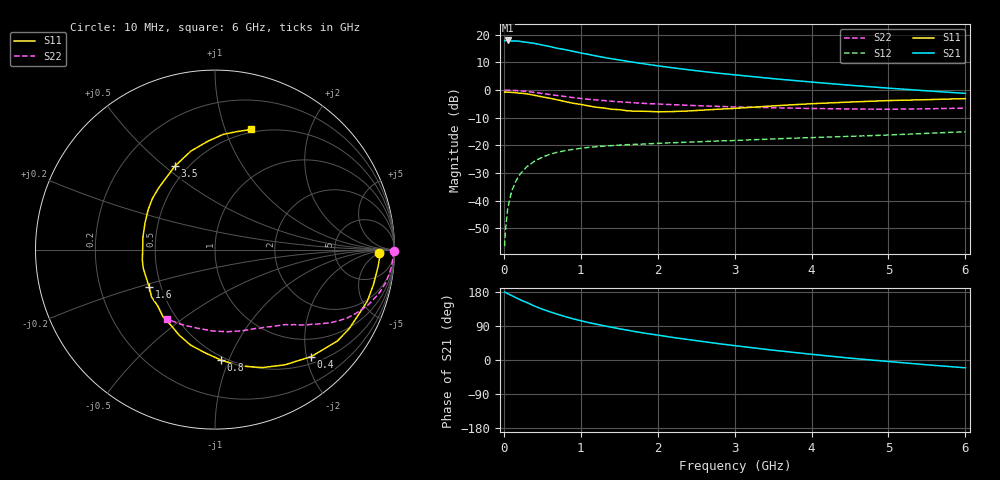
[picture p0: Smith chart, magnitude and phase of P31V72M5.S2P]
! SIEMENS Small Signal Semiconductors
! BFP181
! Si NPN RF Bipolar Junction Transistor in SOT143
! VCE = 1.75 V  IC = 2.5 mA
! Common Emitter S-Parameters:  March  1996
# GHz  S  MA  R  50
!  f  S11  S21  S12  S22
! GHz  MAG  ANG  MAG  ANG  MAG  ANG  MAG  ANG
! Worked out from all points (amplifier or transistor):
!   36 points, 10 MHz to 6 GHz, reference 50 ohm
!   highest |S21| = 17.9 dB at 50 MHz (marker M1)
!   |S21| within 3 dB of that: start of sweep to 729.3 MHz
!   unconditionally stable (mu >= 1): 2.175 GHz to end of sweep
!   at 250 MHz: K = 0.14, MSG = 23.3 dB, |S12| = -29.2 dB
!   at 1.4 GHz: K = 0.73, MSG = 15.7 dB, |S12| = -20.1 dB
!   at 6 GHz: K = 1.14, MAG = 4.7 dB, |S12| = -15.1 dB
!   S11 on the Smith chart (normalised r, x): 10 MHz: 21, -5; 400 MHz: 0.63, -2.09; 800 MHz: 0.47, -0.94; 1.6 GHz: 0.43, -0.22; 3.5 GHz: 0.43, +0.54; 6 GHz: 0.47, +1.23
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0.01  0.9147 -1.3  7.784 179.3  0.0015 84.0  0.9958 -0.5
0.02  0.9192 -2.3  7.827 178.6  0.0028 86.7  0.9929 -1.0
0.05  0.9133 -6.0  7.864 175.0  0.0072 88.6  0.9922 -2.8
0.1  0.9042 -12.4  7.69 170.2  0.0145 80.8  0.9884 -5.6
0.2  0.877 -24.8  7.63 160.2  0.0287 76.0  0.9686 -11.0
0.25  0.8675 -30.7  7.386 155.5  0.0346 72.3  0.9541 -13.6
0.3  0.8508 -36.8  7.279 151.5  0.0411 68.6  0.9394 -15.8
0.4  0.8019 -48.0  6.959 142.1  0.0517 62.9  0.9036 -20.3
0.5  0.7508 -58.8  6.5 134.1  0.0611 57.1  0.8646 -24.1
0.6  0.7079 -68.2  6.102 127.1  0.0689 52.5  0.8287 -27.4
0.8  0.6164 -86.9  5.352 114.3  0.0802 45.0  0.7608 -32.4
0.9  0.5758 -96.0  5.012 108.7  0.0844 41.9  0.7288 -34.4
1.1  0.5166 -112.8  4.403 98.8  0.0915 37.1  0.6794 -37.8
1.3  0.4726 -127.9  3.879 90.4  0.0966 33.2  0.6434 -40.7
1.6  0.4219 -150.3  3.314 78.9  0.1025 29.6  0.6001 -44.2
1.8  0.4129 -165.4  3.007 71.8  0.1052 28.1  0.5752 -46.6
2.2  0.4075 169.9  2.513 59.4  0.1113 25.2  0.5425 -51.7
2.8  0.4502 140.7  2.003 42.9  0.1197 22.5  0.5053 -60.0
3.5  0.5158 115.7  1.603 25.9  0.1304 20.0  0.4774 -71.4
4.5  0.6054 93.7  1.218 4.9  0.1453 16.1  0.4537 -91.7
5.5  0.6689 79.4  0.966 -12.7  0.1645 13.1  0.457 -113.7
6  0.6983 73.4  0.868 -20.6  0.1759 10.6  0.4704 -124.9
